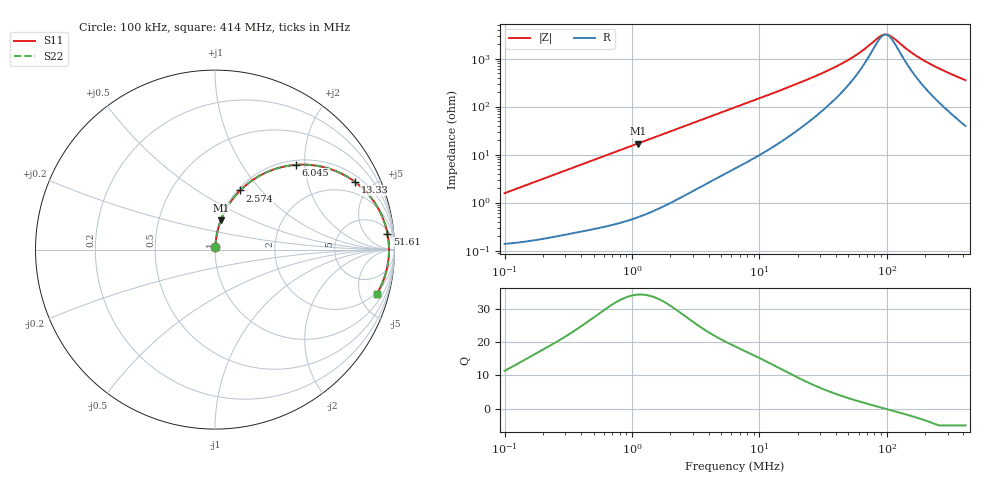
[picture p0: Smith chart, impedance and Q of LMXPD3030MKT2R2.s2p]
! LMXPD3030MKT2R2  S-PARAMETER MODEL  ( General Type )
! Model Generated by TAIYO YUDEN Corporation (http://www.ty-top.com)
! Version 1.0
! TAIYO YUDEN Control No. 191023NI43SB-FBB
! Copyright(c) 2019 TAIYO YUDEN CO.,LTD. All Rights Reserved.
! Product Description (link to TY-COMPAS)
! https://ds.yuden.co.jp/TYCOMPAS/or/detail?pn=LMXPD3030MKT2R2M&u=M
! Products Name : Inductors
! Characteristics :
!  Inductance : 2.2 uH , SRF(min) : 70 MHz , DC Resistance(max) : 0.144 Ohm
!  Rated Current : Saturation :1800 mA , Temp Rise : 1100 mA
!  Case Size : 3.0 x 3.0 / 0.118 x 0.118 [mm/inch] , Thickness : 1.2 / 0.047 [mm/inch]
!  (Conditions: Temperature = 25 degC , DC Bias Current/Voltage = 0A / 0V)
! External Node Assignments :
!  1  o---GGG---o  2
! GND o---------o GND
! Frequency Range : 0.1MHz  -  413.982163MHz  [ 402 STEP ]
# MHz S RI R 50
! Freq[MHz].  S11 Real  S11 Imag  S21 Real  S21 Imag  S12 Real  S12 Imag  S22 Real  S22 Imag
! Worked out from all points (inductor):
!   401 points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, 100 kHz to 414 MHz, reference 50 ohm
!   read as one part in series: L = 2.49 uH near 104.3 kHz
!   highest Q = 34.2 at 1.119 MHz (marker M1), where L = 2.42 uH
!   self-resonance near 97.88 MHz
!   S11 on the Smith chart (normalised r, x): 100 kHz: 1.00, +0.03; 2.574 MHz: 1.03, +0.78; 6.045 MHz: 1.09, +1.80; 13.33 MHz: 1.31, +3.96; 51.61 MHz: 7, +19; 414 MHz: 1.79, -7.06
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0.1  0.00162 0.0156  0.9984 -0.0156  0.9984 -0.0156  0.00162 0.0156
0.403501  0.00629 0.0615  0.9937 -0.0615  0.9937 -0.0615  0.00629 0.0615
1.119244  0.0327 0.1638  0.9673 -0.1638  0.9673 -0.1638  0.0327 0.1638
1.628129  0.0636 0.2293  0.9364 -0.2293  0.9364 -0.2293  0.0636 0.2293
2.574085  0.1398 0.3293  0.8602 -0.3293  0.8602 -0.3293  0.1398 0.3293
3.823222  0.2564 0.4158  0.7436 -0.4158  0.7436 -0.4158  0.2564 0.4158
6.044543  0.4498 0.4721  0.5502 -0.4721  0.5502 -0.4721  0.4498 0.4721
6.434145  0.4789 0.4735  0.5211 -0.4735  0.5211 -0.4735  0.4789 0.4735
8.977803  0.6315 0.4523  0.3685 -0.4523  0.3685 -0.4523  0.6315 0.4523
13.3345  0.7801 0.3769  0.2199 -0.3769  0.2199 -0.3769  0.7801 0.3769
18.22273  0.8602 0.3009  0.1398 -0.3009  0.1398 -0.3009  0.8602 0.3009
25.96183  0.9159 0.2174  0.0841 -0.2174  0.0841 -0.2174  0.9159 0.2174
37.76586  0.9474 0.1418  0.0526 -0.1418  0.0526 -0.1418  0.9474 0.1418
51.61028  0.9608 0.0893  0.0392 -0.0893  0.0392 -0.0893  0.9608 0.0893
64.8938  0.9662 0.0555  0.0338 -0.0555  0.0338 -0.0555  0.9662 0.0555
88.68293  0.9693 0.013  0.0307 -0.013  0.0307 -0.013  0.9693 0.013
96.38509  0.9695 0.00203  0.0305 -0.00203  0.0305 -0.00203  0.9695 0.00203
104.7562  0.9695 -0.00895  0.0305 0.00895  0.0305 0.00895  0.9695 -0.00895
152.3856  0.9659 -0.06  0.0341 0.06  0.0341 0.06  0.9659 -0.06
195.638  0.9597 -0.0978  0.0403 0.0978  0.0403 0.0978  0.9597 -0.0978
278.7244  0.9425 -0.1599  0.0575 0.1599  0.0575 0.1599  0.9425 -0.1599
413.9822  0.9031 -0.2451  0.0969 0.2451  0.0969 0.2451  0.9031 -0.2451
